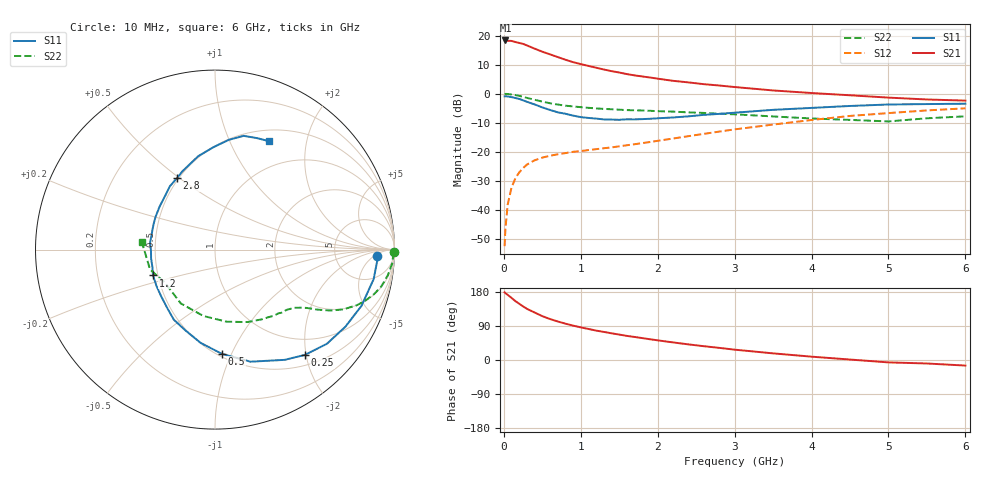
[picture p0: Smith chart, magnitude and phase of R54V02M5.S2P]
! SIEMENS Small Signal Semiconductors
! BFR183
! Si NPN RF Bipolar Junction Transistor in SOT23
! VCE = 4 V  IC = 2.5 mA
! Common Emitter S-Parameters:  May  1996
# GHz  S  MA  R  50
!  f  S11  S21  S12  S22
! GHz  MAG  ANG  MAG  ANG  MAG  ANG  MAG  ANG
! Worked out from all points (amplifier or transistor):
!   36 points, 10 MHz to 6 GHz, reference 50 ohm
!   highest |S21| = 18.3 dB at 20 MHz (marker M1)
!   |S21| within 3 dB of that: start of sweep to 418.1 MHz
!   unconditionally stable (mu >= 1): 1.307 GHz to 2.776 GHz
!   at 250 MHz: K = 0.26, MSG = 21.3 dB, |S12| = -25.5 dB
!   at 1.4 GHz: K = 1.03, MAG = 12.0 dB, |S12| = -18.5 dB
!   at 6 GHz: K = 0.89, MSG = 1.3 dB, |S12| = -5.0 dB
!   S11 on the Smith chart (normalised r, x): 10 MHz: 17, -6; 250 MHz: 0.68, -1.98; 500 MHz: 0.52, -0.92; 1.2 GHz: 0.47, -0.16; 2.8 GHz: 0.49, +0.49; 6 GHz: 0.64, +1.41
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0.01  0.9016 -2.1  8.217 178.6  0.0024 85.9  0.9947 -0.9
0.02  0.9055 -4.2  8.238 176.5  0.0047 85.3  0.9936 -1.7
0.05  0.8992 -10.5  8.134 171.9  0.0124 83.8  0.9903 -4.4
0.1  0.8744 -21.0  8.084 163.9  0.0245 78.9  0.973 -8.5
0.15  0.8439 -30.6  7.746 155.4  0.0352 73.2  0.9485 -12.6
0.25  0.7714 -49.5  7.193 141.4  0.0528 64.2  0.8841 -18.8
0.3  0.7267 -57.7  6.767 135.1  0.0606 61.1  0.849 -21.4
0.4  0.6552 -72.4  5.961 125.3  0.0718 55.4  0.7882 -25.0
0.5  0.5821 -86.2  5.281 115.7  0.0798 51.3  0.7324 -27.6
0.6  0.5264 -98.6  4.756 108.1  0.086 48.8  0.6864 -29.4
0.7  0.4798 -110.0  4.274 101.7  0.091 47.2  0.6523 -30.7
0.8  0.453 -120.4  3.842 95.9  0.0955 46.1  0.6239 -31.7
0.9  0.4209 -129.1  3.493 90.8  0.1004 45.9  0.6049 -32.5
1.1  0.3838 -148.2  3.007 81.9  0.1077 46.6  0.5727 -34.4
1.2  0.3741 -157.4  2.801 77.6  0.1115 47.3  0.5597 -35.4
1.6  0.3637 174.1  2.176 63.6  0.1303 50.7  0.5239 -39.6
2.2  0.3911 142.0  1.666 46.4  0.1699 54.4  0.493 -48.4
2.8  0.4509 118.0  1.385 32.0  0.2235 54.2  0.454 -60.6
3.5  0.5289 100.2  1.139 17.5  0.2953 49.3  0.4073 -80.7
4.5  0.6164 82.8  0.941 1.2  0.4155 37.7  0.3552 -122.4
5.5  0.6643 69.1  0.797 -9.2  0.5168 23.8  0.3785 -163.0
6  0.6741 63.7  0.762 -14.7  0.5618 14.9  0.4091 174.3
